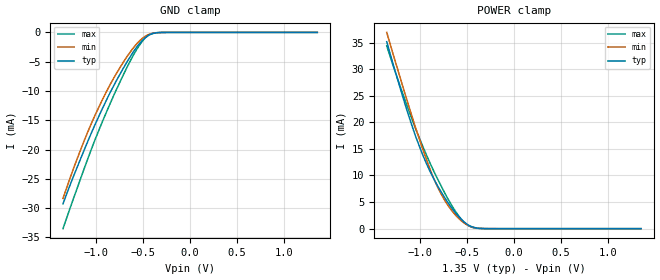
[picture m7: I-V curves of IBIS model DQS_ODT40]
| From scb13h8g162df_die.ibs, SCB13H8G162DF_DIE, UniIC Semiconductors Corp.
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|   Model DQS_ODT40
[Model] DQS_ODT40
Model_type Input
Polarity   Non-Inverting
Enable   Active-High
Vinl =  0.545V
Vinh =  0.805V
C_comp   0.986pF   0.969pF   0.995pF
C_comp_power_clamp   0.234pF   0.227pF   0.238pF
C_comp_gnd_clamp   0.752pF   0.742pF   0.757pF
[Add Submodel]
|  Submodel_name   Mode
DQS_40ohm_ODT   Non-Driving
[Temperature Range]   45.000   95.000   -40.000
[Voltage Range]   1.350V   1.283V   1.425V
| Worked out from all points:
|   GND clamp passes 1 mA (typ) near -0.48 V on its own axis
|   POWER clamp passes 1 mA (typ) near -0.51 V on its own axis
[GND_clamp]
|Voltage   I(typ)   I(min)   I(max)
-1.35V    -29.26mA   -28.34mA   -33.49mA
-1.238V   -24.53mA   -23.21mA   -28.3mA
-1.097V   -18.99mA   -17.39mA   -22.02mA
-1.013V   -15.85mA   -14.25mA   -18.44mA
-872mV    -11.01mA   -9.597mA   -12.98mA
-731mV    -6.729mA   -5.642mA   -7.982mA
-619mV    -3.711mA   -2.975mA   -4.366mA
-534mV    -1.839mA   -1.403mA   -2.088mA
-450mV    -579.7uA   -428.9uA   -569.3uA
-394mV    -185.5uA   -144.2uA   -144.2uA
-281mV    -9.318uA   -9.811uA   -3.103uA
1.35V     0A         0A         0A
[POWER_clamp]
|Voltage   I(typ)   I(min)   I(max)
-1.35V    35.16mA    36.91mA    34.39mA
-1.181V   24.89mA    26.83mA    25.44mA
-1.069V   18.67mA    20.39mA    19.96mA
-956mV    13.38mA    14.37mA    15mA
-872mV    10.11mA    10.36mA    11.63mA
-787mV    7.358mA    7.025mA    8.526mA
-703mV    4.977mA    4.465mA    5.69mA
-619mV    2.933mA    2.534mA    3.219mA
-534mV    1.338mA    1.137mA    1.316mA
-450mV    385.5uA    342uA      284.3uA
-366mV    62.9uA     66.43uA    27.04uA
1.35V     0A         0A         9.135nA
